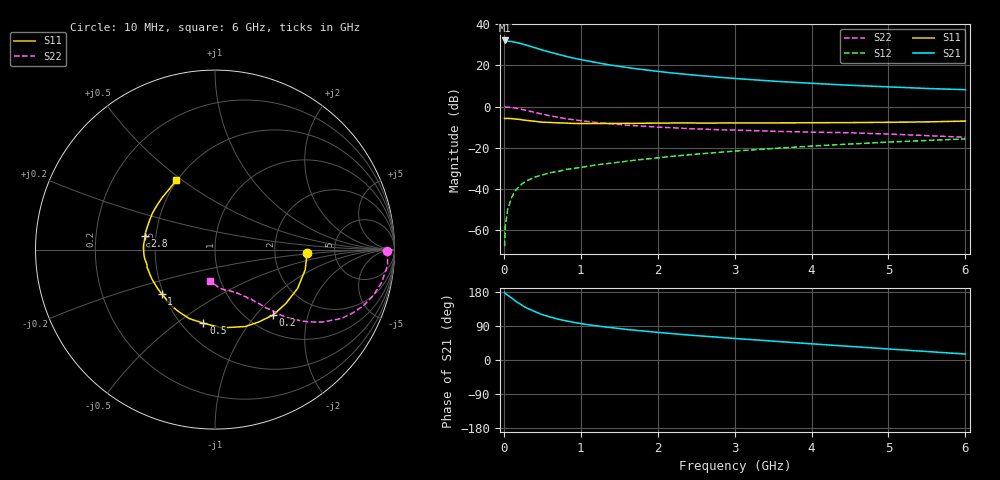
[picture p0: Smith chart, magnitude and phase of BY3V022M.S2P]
! SIEMENS Small Signal Semiconductors
! BFY420
! Si NPN RF SIEGET Grounded Emitter Transistor in MICRO-X
! VCE = 3 V  IC = 22 mA
! Common Emitter S-Parameters:  October  1996
# GHz  S  MA  R  50
!  f  S11  S21  S12  S22
! GHz  MAG  ANG  MAG  ANG  MAG  ANG  MAG  ANG
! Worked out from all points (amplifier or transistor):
!   36 points, 10 MHz to 6 GHz, reference 50 ohm
!   highest |S21| = 32.2 dB at 10 MHz (marker M1)
!   |S21| within 3 dB of that: start of sweep to 357.3 MHz
!   unconditionally stable (mu >= 1): start of sweep to 13.74 MHz; 1.903 GHz to end of sweep
!   at 250 MHz: K = 0.31, MSG = 33.8 dB, |S12| = -37.2 dB
!   at 1.4 GHz: K = 0.92, MSG = 23.8 dB, |S12| = -27.5 dB
!   at 6 GHz: K = 1.06, MAG = 10.4 dB, |S12| = -15.7 dB
!   S11 on the Smith chart (normalised r, x): 10 MHz: 3.11, -0.18; 200 MHz: 1.29, -1.23; 500 MHz: 0.64, -0.63; 1 GHz: 0.49, -0.28; 2.8 GHz: 0.43, +0.08; 6 GHz: 0.49, +0.47
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0.01  0.5143 -2.4  40.59 178.3  0.0004 92.4  0.9593 -0.4
0.02  0.5121 -5.1  40.15 175.4  0.0012 94.2  0.9618 -1.6
0.1  0.5085 -25.3  38.13 163.8  0.006 81.5  0.9468 -11.0
0.15  0.4959 -37.3  36.53 155.5  0.0091 76.3  0.9179 -16.3
0.2  0.4874 -48.5  34.92 149.3  0.0114 72.0  0.8837 -20.8
0.25  0.4707 -59.2  32.91 142.6  0.0138 68.3  0.8412 -25.0
0.3  0.4603 -68.7  30.96 137.0  0.0156 67.0  0.8019 -28.6
0.4  0.4374 -85.2  27.18 128.0  0.0192 62.0  0.7205 -34.1
0.5  0.4152 -98.9  23.69 119.7  0.0217 61.1  0.6516 -38.1
0.6  0.4102 -110.5  21.05 113.6  0.0245 59.9  0.5957 -41.0
0.7  0.4008 -119.7  18.78 108.1  0.0262 59.9  0.5499 -43.4
0.8  0.3971 -128.1  16.81 103.6  0.0293 58.5  0.5104 -45.1
1  0.3864 -140.2  13.87 96.2  0.0329 59.2  0.4534 -47.4
1.1  0.3861 -145.5  12.81 93.1  0.0355 59.3  0.4307 -48.9
1.4  0.3879 -158.1  10.13 85.3  0.042 59.5  0.38 -51.5
1.6  0.3913 -165.1  8.915 80.6  0.0469 59.6  0.3519 -53.3
2.2  0.3979 -180.0  6.526 69.4  0.0617 57.9  0.3041 -58.3
2.8  0.3978 169.0  5.167 59.9  0.0769 55.1  0.2716 -62.9
3.5  0.3989 157.1  4.155 49.8  0.0953 50.8  0.2506 -68.3
4.5  0.4068 142.3  3.294 35.9  0.1224 42.9  0.2302 -76.8
5.5  0.4235 126.5  2.753 22.4  0.1497 33.9  0.1958 -89.7
6  0.4429 119.2  2.572 15.7  0.1633 29.1  0.1786 -98.3
